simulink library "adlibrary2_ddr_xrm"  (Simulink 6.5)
undefined symbols (not defined in the file or in its folder): memsize
libraries: xbsIndex_r4 x30, adlibrary2_ddr_xrm x1

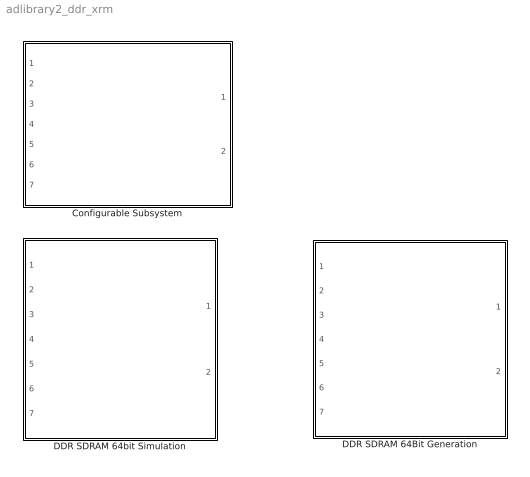
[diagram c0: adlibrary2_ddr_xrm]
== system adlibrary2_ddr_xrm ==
  Configurable Subsystem : Subsystem  Tag=configX  BlockChoice=DDR SDRAM 64bit Simulation
  DDR SDRAM 64Bit Generation : Subsystem
  DDR SDRAM 64bit Simulation : Subsystem  mask{memsize=memsize}
      mask prompts: memsize "Simulation Ram Size (Mb)"

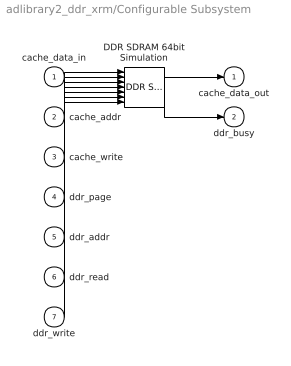
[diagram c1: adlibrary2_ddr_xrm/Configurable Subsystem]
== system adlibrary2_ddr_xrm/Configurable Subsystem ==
  cache_data_in : Inport
  cache_addr : Inport  Port=2
  cache_write : Inport  Port=3
  ddr_page : Inport  Port=4
  ddr_addr : Inport  Port=5
  ddr_read : Inport  Port=6
  ddr_write : Inport  Port=7
  DDR SDRAM 64bit Simulation : adlibrary2_ddr_xrm/DDR SDRAM 64bit Simulation  SystemSampleTime=-1  memsize=memsize
  cache_data_out : Outport
  ddr_busy : Outport  Port=2
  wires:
  cache_data_in/1 -> DDR SDRAM 64bit Simulation/1
  cache_addr/1 -> DDR SDRAM 64bit Simulation/2
  cache_write/1 -> DDR SDRAM 64bit Simulation/3
  ddr_page/1 -> DDR SDRAM 64bit Simulation/4
  ddr_addr/1 -> DDR SDRAM 64bit Simulation/5
  ddr_read/1 -> DDR SDRAM 64bit Simulation/6
  ddr_write/1 -> DDR SDRAM 64bit Simulation/7
  DDR SDRAM 64bit Simulation/1 -> cache_data_out/1
  DDR SDRAM 64bit Simulation/2 -> ddr_busy/1

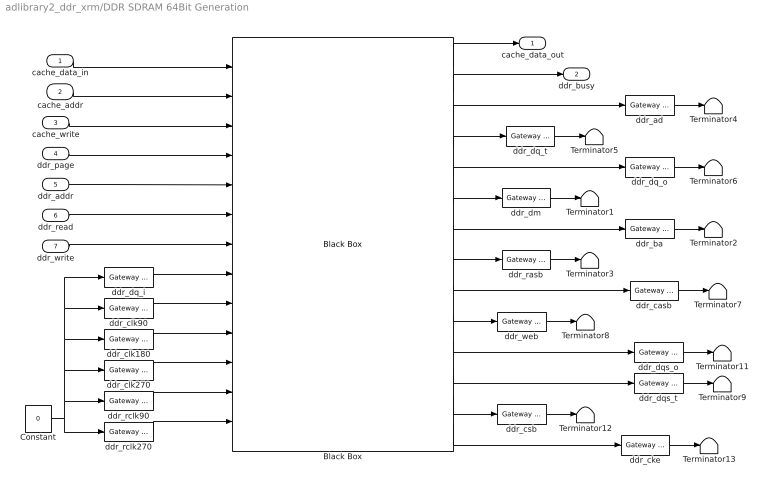
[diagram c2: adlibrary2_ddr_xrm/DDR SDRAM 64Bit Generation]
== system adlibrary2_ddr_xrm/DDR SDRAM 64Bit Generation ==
  cache_data_in : Inport
  cache_addr : Inport  Port=2
  cache_write : Inport  Port=3
  ddr_page : Inport  Port=4
  ddr_addr : Inport  Port=5
  ddr_read : Inport  Port=6
  ddr_write : Inport  Port=7
  Black Box : xbsIndex_r4/Black Box  init_code=ddr64_config  sim_method=Inactive  block_type=blackbox2
  Constant : Constant  Value=0  OutDataType=sfix(16)  ConRadixGroup=Use specified scaling  OutScaling=2^0  SampleTime=inf  FramePeriod=inf
  Terminator{1..9,11..13} (12 alike) : Terminator
  ddr_ad : xbsIndex_r4/Gateway Out  hdl_port=on  timing_constraint=None  locs_specified=off  LOCs={}  block_type=gatewayout
  ddr_ba : xbsIndex_r4/Gateway Out  hdl_port=on  timing_constraint=None  locs_specified=off  LOCs={}  block_type=gatewayout
  ddr_casb : xbsIndex_r4/Gateway Out  hdl_port=on  timing_constraint=None  locs_specified=off  LOCs={}  block_type=gatewayout
  ddr_cke : xbsIndex_r4/Gateway Out  hdl_port=on  timing_constraint=None  locs_specified=off  LOCs={}  block_type=gatewayout
  ddr_clk180 : xbsIndex_r4/Gateway In  arith_type=Boolean  n_bits=64  bin_pt=0  quantization="Round  (unbiased: +/- Inf)"  overflow=Saturate  period=ad_get_simulink_period  dbl_ovrd=off  timing_constraint=None  locs_specified=off  LOCs={}  block_type=gatewayin
  ddr_clk270 : xbsIndex_r4/Gateway In  arith_type=Boolean  n_bits=64  bin_pt=0  quantization="Round  (unbiased: +/- Inf)"  overflow=Saturate  period=ad_get_simulink_period  dbl_ovrd=off  timing_constraint=None  locs_specified=off  LOCs={}  block_type=gatewayin
  ddr_clk90 : xbsIndex_r4/Gateway In  arith_type=Boolean  n_bits=64  bin_pt=0  quantization="Round  (unbiased: +/- Inf)"  overflow=Saturate  period=ad_get_simulink_period  dbl_ovrd=off  timing_constraint=None  locs_specified=off  LOCs={}  block_type=gatewayin
  ddr_csb : xbsIndex_r4/Gateway Out  hdl_port=on  timing_constraint=None  locs_specified=off  LOCs={}  block_type=gatewayout
  ddr_dm : xbsIndex_r4/Gateway Out  hdl_port=on  timing_constraint=None  locs_specified=off  LOCs={}  block_type=gatewayout
  ddr_dq_i : xbsIndex_r4/Gateway In  arith_type=Unsigned  n_bits=64  bin_pt=0  quantization="Round  (unbiased: +/- Inf)"  overflow=Saturate  period=ad_get_simulink_period  dbl_ovrd=off  timing_constraint=None  locs_specified=off  LOCs={}  block_type=gatewayin
  ddr_dq_o : xbsIndex_r4/Gateway Out  hdl_port=on  timing_constraint=None  locs_specified=off  LOCs={}  block_type=gatewayout
  ddr_dq_t : xbsIndex_r4/Gateway Out  hdl_port=on  timing_constraint=None  locs_specified=off  LOCs={}  block_type=gatewayout
  ddr_dqs_o : xbsIndex_r4/Gateway Out  hdl_port=on  timing_constraint=None  locs_specified=off  LOCs={}  block_type=gatewayout
  ddr_dqs_t : xbsIndex_r4/Gateway Out  hdl_port=on  timing_constraint=None  locs_specified=off  LOCs={}  block_type=gatewayout
  ddr_rasb : xbsIndex_r4/Gateway Out  hdl_port=on  timing_constraint=None  locs_specified=off  LOCs={}  block_type=gatewayout
  ddr_rclk270 : xbsIndex_r4/Gateway In  arith_type=Boolean  n_bits=64  bin_pt=0  quantization="Round  (unbiased: +/- Inf)"  overflow=Saturate  period=ad_get_simulink_period  dbl_ovrd=off  timing_constraint=None  locs_specified=off  LOCs={}  block_type=gatewayin
  ddr_rclk90 : xbsIndex_r4/Gateway In  arith_type=Boolean  n_bits=64  bin_pt=0  quantization="Round  (unbiased: +/- Inf)"  overflow=Saturate  period=ad_get_simulink_period  dbl_ovrd=off  timing_constraint=None  locs_specified=off  LOCs={}  block_type=gatewayin
  ddr_web : xbsIndex_r4/Gateway Out  hdl_port=on  timing_constraint=None  locs_specified=off  LOCs={}  block_type=gatewayout
  cache_data_out : Outport
  ddr_busy : Outport  Port=2
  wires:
  Black Box/14 -> ddr_cke/1
  Black Box/13 -> ddr_csb/1
  Black Box/12 -> ddr_dqs_t/1
  Black Box/11 -> ddr_dqs_o/1
  Black Box/10 -> ddr_web/1
  Black Box/9 -> ddr_casb/1
  Black Box/8 -> ddr_rasb/1
  Black Box/7 -> ddr_ba/1
  Black Box/6 -> ddr_dm/1
  Black Box/5 -> ddr_dq_o/1
  Black Box/4 -> ddr_dq_t/1
  Black Box/3 -> ddr_ad/1
  ddr_cke/1 -> Terminator13/1
  ddr_dqs_t/1 -> Terminator9/1
  ddr_rclk270/1 -> Black Box/13
  ddr_rclk90/1 -> Black Box/12
  ddr_clk270/1 -> Black Box/11
  ddr_clk180/1 -> Black Box/10
  ddr_csb/1 -> Terminator12/1
  ddr_dqs_o/1 -> Terminator11/1
  ddr_web/1 -> Terminator8/1
  ddr_casb/1 -> Terminator7/1
  ddr_rasb/1 -> Terminator3/1
  ddr_ba/1 -> Terminator2/1
  ddr_dm/1 -> Terminator1/1
  ddr_dq_o/1 -> Terminator6/1
  ddr_dq_t/1 -> Terminator5/1
  ddr_ad/1 -> Terminator4/1
  Black Box/2 -> ddr_busy/1
  Black Box/1 -> cache_data_out/1
  ddr_write/1 -> Black Box/7
  ddr_read/1 -> Black Box/6
  ddr_addr/1 -> Black Box/5
  ddr_page/1 -> Black Box/4
  cache_write/1 -> Black Box/3
  cache_addr/1 -> Black Box/2
  cache_data_in/1 -> Black Box/1
  ddr_dq_i/1 -> Black Box/8
  ddr_clk90/1 -> Black Box/9
  Constant/1 -> ddr_rclk270/1, ddr_rclk90/1, ddr_clk270/1, ddr_clk180/1, ddr_dq_i/1, ddr_clk90/1

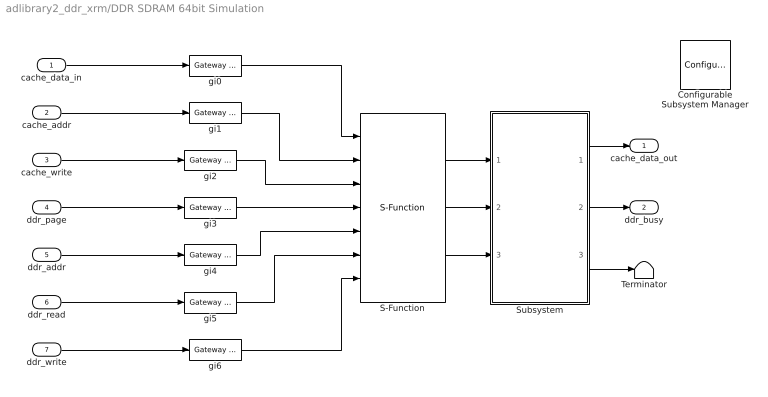
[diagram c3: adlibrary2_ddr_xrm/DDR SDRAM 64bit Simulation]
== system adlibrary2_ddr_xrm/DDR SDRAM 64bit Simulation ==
  cache_data_in : Inport
  cache_addr : Inport  Port=2
  cache_write : Inport  Port=3
  ddr_page : Inport  Port=4
  ddr_addr : Inport  Port=5
  ddr_read : Inport  Port=6
  ddr_write : Inport  Port=7
  Configurable Subsystem Manager : xbsIndex_r4/Configurable Subsystem Manager  Tag=xcfgMgr  block_type=configsubsys
  S-Function : S-Function  FunctionName=ddr64  Parameters=memsize,0
  Subsystem : Subsystem
  Terminator : Terminator
  gi{0..6} (7 alike) : xbsIndex_r4/Gateway Out  hdl_port=off  timing_constraint=None  locs_specified=off  LOCs={}  block_type=gatewayout
  cache_data_out : Outport
  ddr_busy : Outport  Port=2
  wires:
  Subsystem/3(Out3) -> Terminator/1
  Subsystem/2(Out2) -> ddr_busy/1
  Subsystem/1(Out1) -> cache_data_out/1
  S-Function/3 -> Subsystem/3(In3)
  gi6/1 -> S-Function/7
  gi5/1 -> S-Function/6
  gi4/1 -> S-Function/5
  gi3/1 -> S-Function/4
  gi2/1 -> S-Function/3
  gi1/1 -> S-Function/2
  gi0/1 -> S-Function/1
  ddr_write/1 -> gi6/1
  ddr_read/1 -> gi5/1
  ddr_addr/1 -> gi4/1
  ddr_page/1 -> gi3/1
  cache_write/1 -> gi2/1
  cache_addr/1 -> gi1/1
  cache_data_in/1 -> gi0/1
  S-Function/2 -> Subsystem/2(In2)
  S-Function/1 -> Subsystem/1(In1)

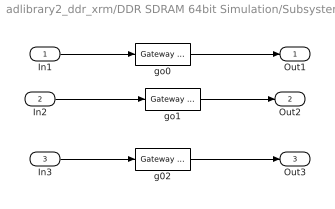
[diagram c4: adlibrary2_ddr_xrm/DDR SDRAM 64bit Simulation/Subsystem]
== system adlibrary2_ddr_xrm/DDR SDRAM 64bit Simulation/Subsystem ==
  In1 : Inport
  In2 : Inport  Port=2
  In3 : Inport  Port=3
  g02 : xbsIndex_r4/Gateway In  arith_type=Unsigned  n_bits=3  bin_pt=0  quantization="Round  (unbiased: +/- Inf)"  overflow=Saturate  period=ad_get_simulink_period  dbl_ovrd=off  timing_constraint=None  locs_specified=off  LOCs={}  block_type=gatewayin
  go0 : xbsIndex_r4/Gateway In  arith_type=Unsigned  n_bits=32  bin_pt=0  quantization="Round  (unbiased: +/- Inf)"  overflow=Saturate  period=ad_get_simulink_period  dbl_ovrd=off  timing_constraint=None  locs_specified=off  LOCs={}  block_type=gatewayin
  go1 : xbsIndex_r4/Gateway In  arith_type=Boolean  n_bits=32  bin_pt=0  quantization="Round  (unbiased: +/- Inf)"  overflow=Saturate  period=ad_get_simulink_period  dbl_ovrd=off  timing_constraint=None  locs_specified=off  LOCs={}  block_type=gatewayin
  Out1 : Outport
  Out2 : Outport  Port=2
  Out3 : Outport  Port=3
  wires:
  g02/1 -> Out3/1
  go1/1 -> Out2/1
  go0/1 -> Out1/1
  In3/1 -> g02/1
  In2/1 -> go1/1
  In1/1 -> go0/1
